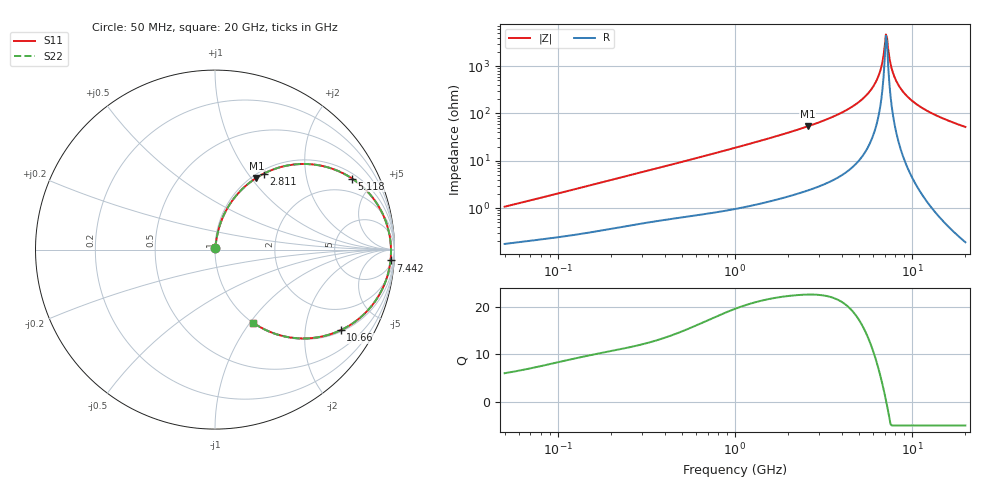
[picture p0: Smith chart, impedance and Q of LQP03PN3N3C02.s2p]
!Murata Part Number: LQP03PN3N3C02
!These Parameters are Measured in Series Mode Connection
!  o--[Z]--o
!Port1  Port2
!  o-------o
!Freq. Start=50[MHz] Stop=20[GHz], 401[Steps]
# Hz S RI R 50
!Freq.(Hz) S11(Real) S11(Imag) S21(Real) S21(Imag) S12(Real) S12(Imag) S22(Real) S22(Imag)
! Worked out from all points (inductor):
!   401 points, 50 MHz to 20 GHz, reference 50 ohm
!   read as one part in series: L = 3.3 nH near 51.52 MHz
!   highest Q = 22.7 at 2.569 GHz (marker M1), where L = 3.3 nH
!   self-resonance near 7.115 GHz
!   S11 on the Smith chart (normalised r, x): 50 MHz: 1.00, +0.02; 2.811 GHz: 1.05, +1.20; 5.118 GHz: 1.22, +3.73; 7.442 GHz: 10, -29; 10.66 GHz: 1.06, -3.09; 20 GHz: 1.00, -1.04
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5e7  0.00186 0.0105  0.9981 -0.0105  0.9981 -0.0105  0.00186 0.0105
1.364002e8  0.00359 0.027  0.9964 -0.027  0.9964 -0.027  0.00359 0.027
3.721004e8  0.0103 0.0698  0.9897 -0.0698  0.9897 -0.0698  0.0103 0.0698
1e9  0.0426 0.1781  0.9574 -0.1781  0.9574 -0.1781  0.0426 0.1781
2.569357e9  0.2307 0.3998  0.7693 -0.3998  0.7693 -0.3998  0.2307 0.3998
2.728004e9  0.258 0.416  0.742 -0.416  0.742 -0.416  0.258 0.416
2.810964e9  0.2728 0.4239  0.7272 -0.4239  0.7272 -0.4239  0.2728 0.4239
4.026975e9  0.5254 0.4762  0.4746 -0.4762  0.4746 -0.4762  0.5254 0.4762
5.117541e9  0.7642 0.3957  0.2358 -0.3957  0.2358 -0.3957  0.7642 0.3957
5.769027e9  0.8779 0.2903  0.1221 -0.2903  0.1221 -0.2903  0.8779 0.2903
6.311513e9  0.9422 0.1809  0.0578 -0.1809  0.0578 -0.1809  0.9422 0.1809
6.601595e9  0.9638 0.1184  0.0362 -0.1184  0.0362 -0.1184  0.9638 0.1184
7.009217e9  0.9791 0.0299  0.0209 -0.0299  0.0209 -0.0299  0.9791 0.0299
7.114996e9  0.9804 0.00733  0.0196 -0.00733  0.0196 -0.00733  0.9804 0.00733
7.331367e9  0.9797 -0.038  0.0203 0.038  0.0203 0.038  0.9797 -0.038
7.442007e9  0.9778 -0.0606  0.0222 0.0606  0.0222 0.0606  0.9778 -0.0606
7.784049e9  0.9659 -0.1273  0.0341 0.1273  0.0341 0.1273  0.9659 -0.1273
8.389408e9  0.9267 -0.2308  0.0733 0.2308  0.0733 0.2308  0.9267 -0.2308
9.316812e9  0.8403 -0.35  0.1597 0.35  0.1597 0.35  0.8403 -0.35
1.066139e10  0.7012 -0.4486  0.2988 0.4486  0.2988 0.4486  0.7012 -0.4486
1.354865e10  0.4621 -0.4942  0.5379 0.4942  0.5379 0.4942  0.4621 -0.4942
2e10  0.2129 -0.4075  0.7871 0.4075  0.7871 0.4075  0.2129 -0.4075
